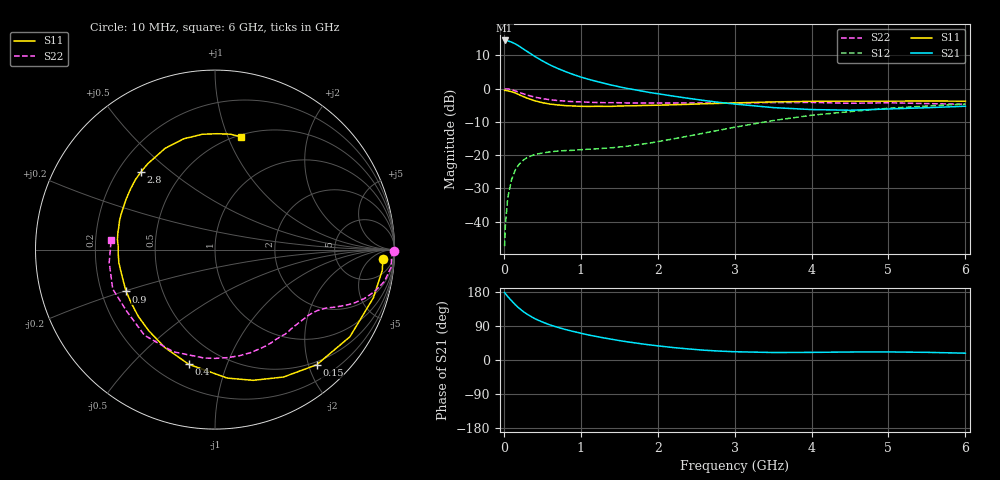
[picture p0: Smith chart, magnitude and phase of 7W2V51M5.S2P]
! Infineon Technologies  Discrete & RF Semiconductors
! BFS17W
! Si NPN RF Bipolar Junction Transistor in SOT323
! VCE = 2.5 V  IC = 1.5 mA
! Common Emitter S-Parameters:  August  1999
# GHz  S  MA  R  50
!  f  S11  S21  S12  S22
! GHz  MAG  ANG  MAG  ANG  MAG  ANG  MAG  ANG
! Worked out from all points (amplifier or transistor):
!   36 points, 10 MHz to 6 GHz, reference 50 ohm
!   highest |S21| = 14.4 dB at 10 MHz (marker M1)
!   |S21| within 3 dB of that: start of sweep to 282.9 MHz
!   unconditionally stable (mu >= 1): 892.4 MHz to end of sweep
!   at 250 MHz: K = 0.32, MSG = 16.7 dB, |S12| = -21.6 dB
!   at 1.4 GHz: K = 1.33, MAG = 6.0 dB, |S12| = -17.8 dB
!   at 6 GHz: K = 1.11, MAG = -2.3 dB, |S12| = -4.7 dB
!   S11 on the Smith chart (normalised r, x): 10 MHz: 17, -15; 150 MHz: 0.45, -2.14; 400 MHz: 0.33, -0.74; 900 MHz: 0.31, -0.20; 2.8 GHz: 0.29, +0.40; 6 GHz: 0.52, +1.11
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0.01  0.9365 -3.3  5.263 178.3  0.0043 86.8  0.9993 -0.6
0.02  0.9392 -7.0  5.255 175.2  0.0089 87.0  0.9846 -2.2
0.05  0.9225 -16.9  5.197 167.7  0.0225 80.5  0.9864 -5.6
0.1  0.8947 -32.9  4.972 156.5  0.0427 72.0  0.9608 -10.6
0.15  0.8558 -48.6  4.668 145.6  0.0602 63.3  0.9185 -14.8
0.2  0.8062 -61.7  4.32 136.3  0.0735 57.6  0.8764 -18.1
0.25  0.7589 -73.7  3.945 128.2  0.0834 51.3  0.8352 -20.7
0.3  0.719 -84.6  3.617 121.2  0.0916 47.6  0.8008 -22.6
0.4  0.6555 -102.9  3.044 109.4  0.1019 41.3  0.7434 -25.5
0.5  0.6128 -117.2  2.604 100.3  0.1075 37.5  0.7053 -27.4
0.6  0.5836 -129.2  2.258 92.6  0.1119 35.6  0.6786 -29.3
0.7  0.5667 -139.0  2.001 86.3  0.1153 34.9  0.6603 -31.2
0.9  0.5474 -154.8  1.626 75.4  0.1181 34.9  0.635 -35.4
1.1  0.5384 -167.4  1.377 66.0  0.1227 36.7  0.6226 -40.0
1.4  0.5392 178.3  1.124 54.8  0.1289 41.9  0.6131 -47.6
1.6  0.5494 169.9  1.004 48.1  0.136 45.7  0.6067 -53.2
2.2  0.5695 150.3  0.77 32.9  0.1751 56.6  0.6073 -71.0
2.8  0.5981 133.5  0.619 23.5  0.2368 60.5  0.6061 -89.9
3.5  0.6291 116.2  0.517 19.8  0.3303 57.9  0.6148 -112.1
4.5  0.6464 96.3  0.472 21.1  0.45 46.1  0.5999 -145.1
5.5  0.6486 82.5  0.515 20.2  0.546 33.6  0.5938 -173.1
6  0.6456 77.2  0.542 18.0  0.5834 27.7  0.5808 174.6
